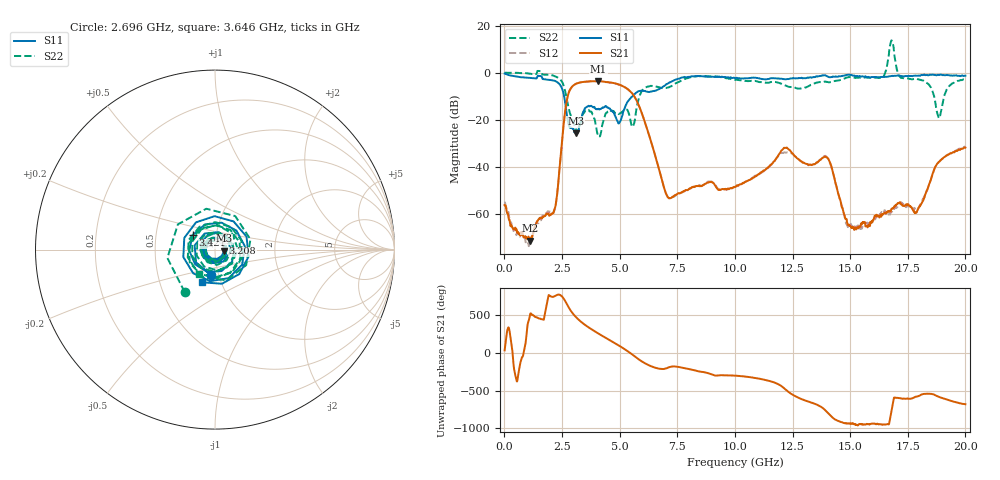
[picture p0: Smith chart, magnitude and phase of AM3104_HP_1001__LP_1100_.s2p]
!Created with skrf (http://scikit-rf.org).
# Hz S RI R 50.0
!freq ReS11 ImS11 ReS21 ImS21 ReS12 ImS12 ReS22 ImS22
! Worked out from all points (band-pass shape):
!   1601 points, 10 MHz to 20 GHz, reference 50 ohm
!   highest |S21| = -3.64 dB at 4.083 GHz (marker M1); lowest = -71.4 dB at 1.097 GHz (marker M2)
!   |S21| within 3 dB of the highest: 2.885 GHz to 5.295 GHz (2.41 GHz wide, 58.9 % of centre)
!   lowest |S11| = -25.8 dB at 3.096 GHz (marker M3), VSWR 1.11, Z = 55.4 - j0.664 ohm
!   |S11| at or under -10 dB: 2.59 GHz to 5.563 GHz (2.973 GHz wide, 72.9 % of centre)
!   |S22| runs from -27.1 to 13.6 dB; largest |S21 - S12| = 0.058
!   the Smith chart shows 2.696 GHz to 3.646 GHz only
!   S11 on the Smith chart (normalised r, x): 2.696 GHz: 0.92, -0.26; 3.208 GHz: 1.09, +0.08; 3.421 GHz: 0.77, +0.13; 3.646 GHz: 0.81, -0.31
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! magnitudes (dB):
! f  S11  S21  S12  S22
! 10 MHz  -0.4  -56.3  -55.2  -0.1
! 1.097 GHz  -2.3  -71.4  -72.7  -0.5
! 2.171 GHz  -3.5  -58.0  -58.6  -1.5
! 2.696 GHz  -17.0  -12.5  -12.5  -10.7
! 3.096 GHz  -25.8  -4.8  -4.8  -24.3
! 3.208 GHz  -25.0  -4.4  -4.4  -24.7
! 3.346 GHz  -19.4  -4.1  -4.1  -19.8
! 3.421 GHz  -16.6  -4.0  -4.0  -17.4
! 3.646 GHz  -14.1  -3.8  -3.9  -15.9
! 4.083 GHz  -15.4  -3.6  -3.7  -27.0
! 5.595 GHz  -9.6  -9.5  -9.5  -22.4
! 6.682 GHz  -7.2  -40.1  -40.0  -6.1
! 7.169 GHz  -4.1  -53.3  -53.2  -6.1
! 10.01 GHz  -2.4  -48.6  -48.6  -3.1
! 12.17 GHz  -2.8  -32.0  -33.9  -5.4
! 13.34 GHz  -2.1  -39.2  -39.2  -5.1
! 14.05 GHz  -1.8  -36.6  -36.7  -4.1
! 15.08 GHz  -1.1  -65.6  -65.2  -2.0
! 16.68 GHz  -1.6  -59.1  -60.2  7.3
! 17.89 GHz  -1.3  -59.4  -58.1  -2.7
! 18.84 GHz  -1.0  -38.0  -38.2  -19.1
! 20 GHz  -1.3  -31.9  -31.4  -2.7
